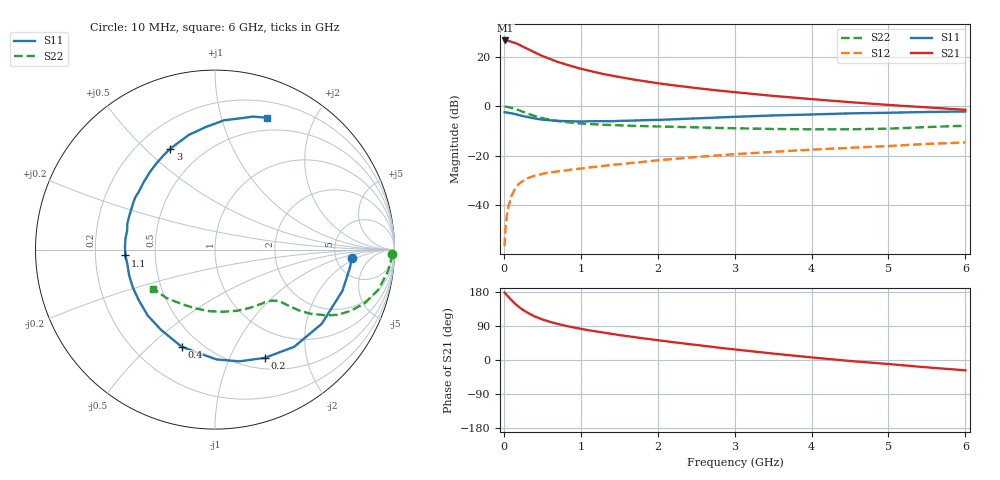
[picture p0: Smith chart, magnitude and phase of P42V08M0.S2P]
! SIEMENS Small Signal Semiconductors
! BFP182
! Si NPN RF Bipolar Junction Transistor in SOT143
! VCE = 2 V  IC = 8 mA
! Common Emitter S-Parameters:  March  1996
# GHz  S  MA  R  50
!  f  S11  S21  S12  S22
! GHz  MAG  ANG  MAG  ANG  MAG  ANG  MAG  ANG
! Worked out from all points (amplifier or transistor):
!   36 points, 10 MHz to 6 GHz, reference 50 ohm
!   highest |S21| = 26.6 dB at 20 MHz (marker M1)
!   |S21| within 3 dB of that: start of sweep to 280.8 MHz
!   unconditionally stable (mu >= 1): 1.248 GHz to 5.406 GHz
!   at 250 MHz: K = 0.29, MSG = 27.1 dB, |S12| = -30.1 dB
!   at 1.4 GHz: K = 1.06, MAG = 16.6 dB, |S12| = -23.7 dB
!   at 6 GHz: K = 0.94, MSG = 6.6 dB, |S12| = -14.6 dB
!   lowest NFmin = 1.40 dB at 450 MHz
!   S11 on the Smith chart (normalised r, x): 10 MHz: 7.08, -1.58; 200 MHz: 0.63, -1.36; 400 MHz: 0.40, -0.64; 1.1 GHz: 0.33, -0.03; 3 GHz: 0.33, +0.60; 6 GHz: 0.36, +1.40
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0.01  0.7631 -3.5  21.29 177.8  0.0015 87.6  0.9842 -1.4
0.02  0.7593 -7.2  21.46 175.9  0.0034 81.0  0.9849 -2.9
0.05  0.7463 -17.9  21.34 168.6  0.0084 83.6  0.9714 -7.2
0.1  0.7242 -34.8  20.11 158.0  0.0156 72.2  0.9363 -13.9
0.15  0.6983 -50.9  19.01 147.9  0.0222 65.4  0.8856 -19.7
0.2  0.6637 -65.3  17.6 139.3  0.0277 60.3  0.8293 -24.3
0.25  0.6375 -77.6  16 132.0  0.0312 55.7  0.7757 -27.9
0.3  0.6119 -89.2  14.71 125.8  0.0351 51.8  0.7245 -30.4
0.4  0.5728 -108.8  12.36 115.0  0.0398 46.6  0.641 -33.9
0.5  0.5388 -123.9  10.43 107.1  0.0434 43.7  0.581 -35.8
0.6  0.5248 -135.7  9.088 100.7  0.0464 41.8  0.5389 -36.8
0.7  0.5094 -146.8  7.921 95.2  0.0485 41.0  0.5076 -37.5
0.9  0.4998 -163.0  6.379 86.3  0.0535 40.7  0.4645 -38.6
1.1  0.5002 -176.3  5.292 78.6  0.0583 40.6  0.4414 -40.2
1.5  0.5094 163.5  3.926 65.8  0.0678 41.0  0.4142 -44.1
1.8  0.5245 150.4  3.276 57.5  0.0755 41.2  0.4008 -48.0
2.2  0.547 136.5  2.671 47.1  0.0864 40.2  0.3869 -54.4
3  0.615 113.9  1.939 27.9  0.1082 36.4  0.3619 -70.3
3.5  0.6557 102.8  1.629 17.0  0.1206 33.1  0.3496 -82.0
4.5  0.7227 85.9  1.217 -2.6  0.1458 26.3  0.3451 -108.4
5.5  0.7706 74.1  0.956 -19.4  0.1748 19.5  0.3819 -135.0
6  0.7892 68.6  0.853 -27.2  0.1863 14.7  0.407 -147.6
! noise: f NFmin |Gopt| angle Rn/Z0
0.45  1.4  0.26  41  0.29
0.9  1.5  0.25  83  0.23
1.8  2  0.21  162  0.2
